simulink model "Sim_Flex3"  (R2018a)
settings: Solver=VariableStepAuto  StartTime=0.0  StopTime=20.0  RelTol=1e-3
InitFcn:
  | init
StopFcn:
  | pl
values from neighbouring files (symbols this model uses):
  d2r = 1/r2d    (= 0.0174532925199)    [init.m]
undefined symbols (not defined in the file or in its folder): Ac, Bc, Cc, Dc

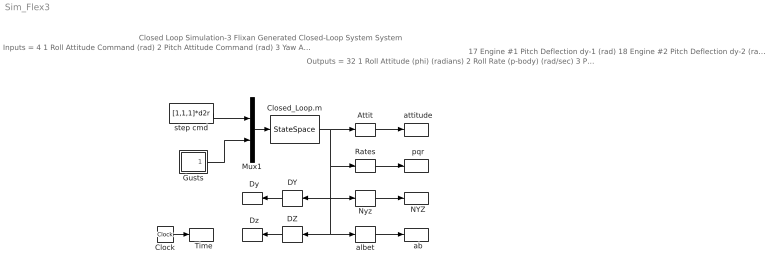
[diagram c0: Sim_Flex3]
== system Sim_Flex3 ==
  note: Outputs = 32 1 Roll Attitude (phi) (radians) 2 Roll Rate (p-body) (rad/sec) 3 Pitch Attitude (thet) (radians) 4 Pitch Rate (q-body) (rad/sec) 5 Yaw Attitude (psi) (radians) 6 Yaw Rate (r-body) (rad/sec) 7 Angle of attack, alfa, (radian) 8 Angle of sideslip, beta, (radian) 9 Change in Altitude, delta-h, (feet) 10 Forward Acceleration (V-dot) (ft/sec) 11 Cross Range Velocity (Vcr) (ft/sec) 12 Rate-Gyro # 1, Roll Rate (Body) (rad/sec) 13 Rate-Gyro # 2, Pitch Rate (Body) (rad/sec) 14 Rate-Gyro # 3, Yaw Rate (Body) (rad/sec) 15 Accelerom # 1, (along Y), (ft/sec^2) Translat. Accelerat. 16 Accelerom # 2, (along Z), (ft/sec^2) Translat. Accelerat.
  note: Inputs = 4 1 Roll Attitude Command (rad) 2 Pitch Attitude Command (rad) 3 Yaw Attitude Command (rad) 4 Wind-Gust Velocity (feet/sec)
  note: 17 Engine #1 Pitch Deflection dy-1 (rad) 18 Engine #2 Pitch Deflection dy-2 (rad) 19 Engine #3 Pitch Deflection dy-3 (rad) 20 Engine #4 Pitch Deflection dy-4 (rad) 21 Engine #5 Pitch Deflection dy-5 (rad) 22 Engine #6 Pitch Deflection dy-6 (rad) 23 Engine #7 Pitch Deflection dy-7 (rad) 24 Engine #8 Pitch Deflection dy-8 (rad) 25 Engine #1 Yaw Deflection dz-1 (rad) 26 Engine #2 Yaw Deflection dz-2 (rad) 27 Engine #3 Yaw Deflection dz-3 (rad) 28 Engine #4 Yaw Deflection dz-4 (rad) 29 Engine #5 Yaw Deflection dz-5 (rad) 30 Engine #6 Yaw Deflection dz-6 (rad) 31 Engine #7 Yaw Deflection dz-7 (rad) 32 Engine #8 Yaw Deflection dz-8 (rad)
  note: Closed Loop Simulation-3 Flixan Generated Closed-Loop System System
  "  Dy" : ToWorkspace  VariableName=DY  SampleTime=-1
  "  Dz" : ToWorkspace  VariableName=DZ  SampleTime=-1
  "  NYZ" : ToWorkspace  VariableName=Nyz  SampleTime=-1
  "  Time" : ToWorkspace  VariableName=tim  SampleTime=-1
  "  ab" : ToWorkspace  VariableName=albet  SampleTime=-1
  "  attitude" : ToWorkspace  VariableName=atti  SampleTime=-1
  "  pqr" : ToWorkspace  VariableName=pqr  SampleTime=-1
  Attit : Selector  InputPortWidth=32  IndexOptions=Index vector (dialog)  Indices=[1,3,5]  OutputSizes=1
  Clock : Clock
  Closed_Loop.m : StateSpace  A=Ac  B=Bc  C=Cc  D=Dc  InitialCondition=0
  DY : Selector  InputPortWidth=32  IndexOptions=Index vector (dialog)  Indices=[17:24]  OutputSizes=1
  DZ : Selector  InputPortWidth=32  IndexOptions=Index vector (dialog)  Indices=[25:32]  OutputSizes=1
  Gusts : Subsystem
  Mux1 : Mux  Inputs=[3, 1]
  Nyz : Selector  InputPortWidth=32  IndexOptions=Index vector (dialog)  Indices=[15,16]  OutputSizes=1
  Rates : Selector  InputPortWidth=32  IndexOptions=Index vector (dialog)  Indices=[12:14]  OutputSizes=1
  albet : Selector  InputPortWidth=32  IndexOptions=Index vector (dialog)  Indices=[7,8]  OutputSizes=1
  step cmd : Constant  Value=[1,1,1]*d2r
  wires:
  step cmd/1 -> Mux1/1
  Attit/1 -> "  attitude"/1
  albet/1 -> "  ab"/1
  Clock/1 -> "  Time"/1
  Nyz/1 -> "  NYZ"/1
  Rates/1 -> "  pqr"/1
  Mux1/1 -> Closed_Loop.m/1
  Closed_Loop.m/1 -> DY/1, albet/1, DZ/1, Nyz/1, Rates/1, Attit/1
  DZ/1 -> "  Dz"/1
  DY/1 -> "  Dy"/1
  Gusts/1(Wgst) -> Mux1/2

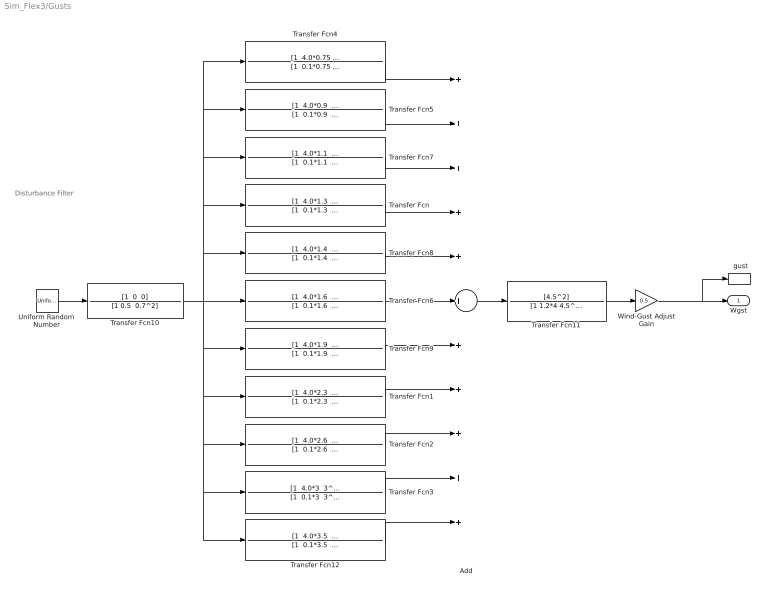
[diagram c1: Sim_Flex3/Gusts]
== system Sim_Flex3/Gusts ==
  note: Disturbance Filter
  "  gust" : ToWorkspace  VariableName=Wgst  SampleTime=-1
  Add : Sum  Inputs=+++++++++++
  Transfer Fcn : TransferFcn  Numerator="[1  4.0*1.3  1.3^2]"  Denominator="[1  0.1*1.3  1.3^2]"
  Transfer Fcn1 : TransferFcn  Numerator="[1  4.0*2.3  2.3^2]"  Denominator="[1  0.1*2.3  2.3^2]"
  Transfer Fcn10 : TransferFcn  Numerator="[1  0  0]"  Denominator="[1 0.5  0.7^2]"
  Transfer Fcn11 : TransferFcn  Numerator=[4.5^2]  Denominator=[1 1.2*4 4.5^2]
  Transfer Fcn12 : TransferFcn  Numerator="[1  4.0*3.5  3.5^2]"  Denominator="[1  0.1*3.5  3.5^2]"
  Transfer Fcn2 : TransferFcn  Numerator="[1  4.0*2.6  2.6^2]"  Denominator="[1  0.1*2.6  2.6^2]"
  Transfer Fcn3 : TransferFcn  Numerator="[1  4.0*3  3^2]"  Denominator="[1  0.1*3  3^2]"
  Transfer Fcn4 : TransferFcn  Numerator="[1  4.0*0.75  0.75^2]"  Denominator="[1  0.1*0.75  0.75^2]"
  Transfer Fcn5 : TransferFcn  Numerator="[1  4.0*0.9  0.9^2]"  Denominator="[1  0.1*0.9  0.9^2]"
  Transfer Fcn6 : TransferFcn  Numerator="[1  4.0*1.6  1.6^2]"  Denominator="[1  0.1*1.6  1.6^2]"
  Transfer Fcn7 : TransferFcn  Numerator="[1  4.0*1.1  1.1^2]"  Denominator="[1  0.1*1.1  1.1^2]"
  Transfer Fcn8 : TransferFcn  Numerator="[1  4.0*1.4  1.4^2]"  Denominator="[1  0.1*1.4  1.4^2]"
  Transfer Fcn9 : TransferFcn  Numerator="[1  4.0*1.9  1.9^2]"  Denominator="[1  0.1*1.9  1.9^2]"
  Uniform Random Number : UniformRandomNumber  SampleTime=0.1
  Wind-Gust Adjust Gain : Gain  Gain=0.5
  Wgst : Outport
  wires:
  Uniform Random Number/1 -> Transfer Fcn10/1
  Transfer Fcn12/1 -> Add/11
  Transfer Fcn3/1 -> Add/10
  Transfer Fcn11/1 -> Wind-Gust Adjust Gain/1
  Transfer Fcn6/1 -> Add/6
  Transfer Fcn5/1 -> Add/2
  Transfer Fcn4/1 -> Add/1
  Transfer Fcn/1 -> Add/4
  Add/1 -> Transfer Fcn11/1
  Transfer Fcn7/1 -> Add/3
  Transfer Fcn1/1 -> Add/8
  Transfer Fcn10/1 -> Transfer Fcn6/1, Transfer Fcn5/1, Transfer Fcn4/1, Transfer Fcn7/1, Transfer Fcn/1, Transfer Fcn8/1, Transfer Fcn1/1, Transfer Fcn2/1, Transfer Fcn12/1, Transfer Fcn3/1, Transfer Fcn9/1
  Transfer Fcn2/1 -> Add/9
  Transfer Fcn8/1 -> Add/5
  Transfer Fcn9/1 -> Add/7
  Wind-Gust Adjust Gain/1 -> "  gust"/1, Wgst/1
